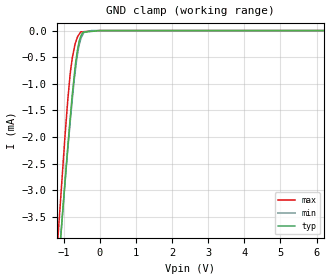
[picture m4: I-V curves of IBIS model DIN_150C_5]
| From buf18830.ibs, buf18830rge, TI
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[Model]   DIN_150C_5   |Rload to VDD = 1k ohms
Model_type   Input
|Signals
Vinl = 1.5
Vinh = 3.5
|   typ   min   max
|   (Fast PVT)   (Nom PVT)   (slow PVT)
C_comp   5.4311E-13   5.3466E-13   6.9030E-13
| Where   Nom PVT is  Nominal Process, 5.0V, 92C
|   Fast PVT is Strong Process, 5.5V, -40C
|   Slow PVT is Weak Process, 4.5V, 150C
[Model Spec]   |5V model
Vinl   1.5   1.35   1.65
Vinh   3.5   3.15   3.85
|Vinl = 0.3 X DVDD
|Vinh = 0.7 X DVDD
[Voltage Range]   5   4.5   5.5
|Operating Temperature   27   85   -40
[Temperature Range]   92   150   -40
[Power Clamp Reference]   5   4.5   5.5
[GND Clamp Reference]   0   0   0
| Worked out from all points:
|   GND clamp passes 1 mA (typ) near -0.73 V on its own axis
[GND Clamp]
|   Voltage   I(typ)   I(min)   I(max)
-5V       -41.9mA    -39.83mA   -45.76mA
-1.228V   -5.205mA   -5.098mA   -4.548mA
-1.037V   -3.469mA   -3.476mA   -2.683mA
-891.4mV  -2.21mA    -2.259mA   -1.334mA
-803.4mV  -1.511mA   -1.575mA   -710.1uA
-757.6mV  -1.163mA   -1.254mA   -490.9uA
-666.2mV  -577.7uA   -678.4uA   -212.5uA
-583.7mV  -237.9uA   -302.1uA   -79.93uA
-529.3mV  -106.7uA   -158.5uA   -24.67uA
-435.3mV  -29.27uA   -31.93uA   -20.14uA
-236.4mV  -15.89uA   -230.4nA   -10.56uA
9.985V    0A         0A         0A
|DVDD = 5V
[POWER Clamp]
|   SCR cell for ESD function. Effects occurr above VDD x 2
|   Voltage   I(typ)   I(min)   I(max)
-5V       0A         0A         0A
0V        0A         0A         0A
10V       0A         0A         0A
